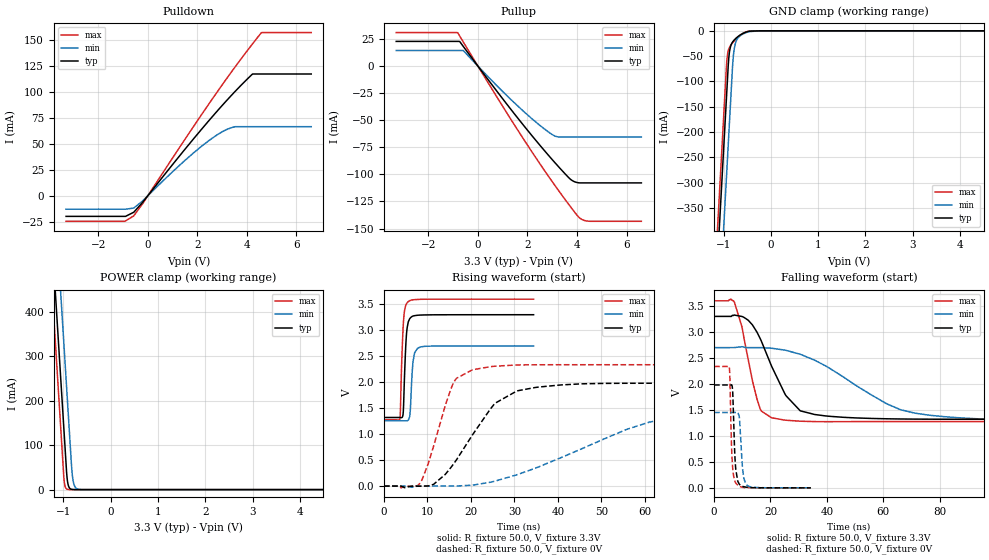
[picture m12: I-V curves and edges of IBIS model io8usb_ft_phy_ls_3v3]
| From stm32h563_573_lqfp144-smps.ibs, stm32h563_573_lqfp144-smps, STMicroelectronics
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[Model]   io8usb_ft_phy_ls_3v3
Model_type I/O
Polarity   Non-Inverting
Enable   Active-Low
| CAP_THRESHOLD on pad DPFT is "UDTCAPC" :
| Rising=20.0% of vddiom   Falling=80.0% of vddiom
| C_comp min and max val. don't necessarily correlate with the min and max pvt
| but are the smallest and greatest pad capacitance found.
| var   typ   min   max
C_comp   8.88570pF  8.80266pF  8.92058pF
|C_comp_pullup   6.10735pF  5.78805pF  5.62765pF
|C_comp_pulldown   2.77835pF  3.01461pF  3.29293pF
Vinl = 1.35V
Vinh = 1.8V
Vmeas = 1.65V   | Reference voltage for timing measurements
Cref  = 50.0pF   | Timing specification test load capacitance value
Rref  = 1.0MOhm   | Timing specification test load resistance value
Vref  = 1.815V   | Timing specification test load voltage
[Model Spec]
| TIME_THRESHOLD on pin ZIUSBPV11 is "CMOS" :
| Rising=40.0% of vdd   Falling=60.0% of vdd
Vinl 1.31380V 1.08880V 1.42380V
Vinh 1.79320V 1.51020V 1.91620V
| variable   typ   min   max
[Temperature Range] 25.0 125.0 -40.0
| variable   typ   min   max
[Voltage Range] 3.3V 2.7V 3.6V
| variable   typ   min   max
[POWER Clamp Reference] 3.3V 2.7V 3.6V
| variable   typ   min   max
[GND Clamp Reference] 0V 0V 0V
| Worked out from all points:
|   slope of the pulldown table from 0 to 0.495 V, typ, clamps not added: 33.1 ohm
|   slope of the pullup table from 0 to 0.495 V, typ, clamps not added: 32.9 ohm
|   GND clamp passes 1 mA (typ) near -0.46 V on its own axis
|   POWER clamp passes 1 mA (typ) near -0.84 V on its own axis
|   rising waveform, R_fixture 50.0, V_fixture 3.3V: 20-80 % time 589ps typ, 600ps min, 595ps max; typ from 1.32 V to 3.3 V
|   falling waveform, R_fixture 50.0, V_fixture 3.3V: 20-80 % time 10.4ns typ, 27.1ns min, 5.39ns max; typ from 3.3 V to 1.32 V
|   rising waveform, R_fixture 50.0, V_fixture 0V: 20-80 % time 9.68ns typ, 25.4ns min, 5.08ns max; typ from 0 V to 1.98 V
|   falling waveform, R_fixture 50.0, V_fixture 0V: 20-80 % time 860ps typ, 1.08ns min, 778ps max; typ from 1.98 V to 0 V
[POWER Clamp]
-3.3V     4.068A     4.259A     3.957A
-1.25V    582.8mA    774.2mA    471.5mA
-1.16V    429.8mA    621.2mA    318.5mA
-1.05V    242.8mA    434.2mA    131.5mA
-980mV    123.8mA    315.2mA    17.95mA
-960mV    89.81mA    281.2mA    6.634mA
-920mV    26.3mA     213.2mA    906uA
-880mV    5.543mA    145.2mA    123.7uA
-810mV    363.5uA    33.6mA     3.798uA
-770mV    76.63uA    10.47mA    519.9nA
-690mV    3.411uA    1.017mA    10.89nA
6.6V      0A         0A         0A
[GND Clamp]
-3.3V     -4.147A    -4.304A    -4.084A
-1.25V    -662.3mA   -818.9mA   -599mA
-940mV    -135.3mA   -291.9mA   -71.97mA
-910mV    -84.3mA    -240.9mA   -43.19mA
-890mV    -54.53mA   -206.9mA   -36.04mA
-870mV    -38.95mA   -172.9mA   -31.83mA
-810mV    -22.29mA   -70.86mA   -23.78mA
-780mV    -18.66mA   -39.68mA   -20.49mA
-750mV    -15.77mA   -25.18mA   -17.46mA
-710mV    -12.47mA   -16.15mA   -13.75mA
-540mV    -3.025mA   -4.157mA   -2.753mA
6.6V      24.07nA    4.253uA    975.9pA
| variable   typ   min   max
[Pullup Reference] 3.3V 2.7V 3.6V
| variable   typ   min   max
[Pulldown Reference] 0V 0V 0V
[Pullup]
-3.3V     22.83mA    14.39mA    31mA
-820mV    22.83mA    14.39mA    31mA
-740mV    22.83mA    14.39mA    27.95mA
-590mV    18.16mA    14.39mA    22.24mA
1.32V     -39.61mA   -30.57mA   -48.77mA
2.85V     -82.4mA    -60.84mA   -101.8mA
3.19V     -91.23mA   -65.16mA   -112.8mA
3.7V      -103.7mA   -65.39mA   -128.7mA
4.06V     -107.7mA   -65.39mA   -139.2mA
4.22V     -107.9mA   -65.39mA   -141.9mA
4.51V     -107.9mA   -65.39mA   -143.3mA
6.6V      -107.9mA   -65.39mA   -143.3mA
[Pulldown]
-3.3V     -19.88mA   -12.95mA   -24.65mA
-940mV    -19.88mA   -12.95mA   -24.65mA
-570mV    -15.96mA   -11.9mA    -19.44mA
-220mV    -6.69mA    -5.247mA   -8.037mA
1.48V     44.27mA    33.69mA    53.76mA
2.17V     64.17mA    47.77mA    78.28mA
2.8V      81.66mA    58.79mA    100.1mA
3.19V     92.07mA    63.96mA    113.3mA
3.51V     100.3mA    66.56mA    123.9mA
4.23V     117.5mA    66.66mA    146.6mA
4.59V     117.5mA    66.66mA    157.5mA
6.6V      117.5mA    66.66mA    157.5mA
[Ramp]
dV/dt_r 1.18821V/9.67363ns 870.42399mV/24.97673ns 1.40193V/5.07203ns
dV/dt_f 1.18779V/10.0041ns 865.87422mV/26.69286ns 1.3938V/5.29566ns
R_load = 50.0
| Removed startup time: 0s 0s 0s  .
| Removed end time: 34.4ns.
[Rising Waveform]
R_fixture   = 50.0
V_fixture   = 3.3V
V_fixture_min = 2.7V
V_fixture_max = 3.6V
0s        1.32V      1.257V     1.277V
3.65ns    1.32V      1.257V     1.288V
3.75ns    1.32V      1.257V     1.376V
4.5ns     1.521V     1.257V     3.181V
5.05ns    2.754V     1.257V     3.486V
5.6ns     3.163V     1.268V     3.553V
6ns       3.232V     1.396V     3.573V
6.7ns     3.275V     2.404V     3.587V
7.75ns    3.29V      2.656V     3.594V
34.4ns    3.3V       2.7V       3.6V
| Removed startup time: 0s 0s 0s  .
| Removed end time: 249.35ns.
[Falling Waveform]
R_fixture   = 50.0
V_fixture   = 3.3V
V_fixture_min = 2.7V
V_fixture_max = 3.6V
0s        3.3V       2.7V       3.6V
7.2ns     3.326V     2.7V       3.575V
9.9ns     3.298V     2.717V     3.096V
12.2ns    3.221V     2.699V     2.444V
16.75ns   2.826V     2.699V     1.478V
25ns      1.821V     2.652V     1.304V
35.65ns   1.412V     2.458V     1.276V
61.1ns    1.33V      1.621V     1.277V
76.35ns   1.322V     1.398V     1.277V
249.3ns   1.32V      1.257V     1.277V
| Removed startup time: 0s 0s 0s  .
| Removed end time: 249.4ns.
[Rising Waveform]
R_fixture   = 50.0
V_fixture   = 0V
V_fixture_min = 0V
V_fixture_max = 0V
0s        24.82nV    1.065uV    39.76nV
8.1ns     -1.878mV   -1.788mV   37.66mV
11.4ns    31.98mV    -774.9uV   764.2mV
16.2ns    449.3mV    472.3uV    2.017V
24.4ns    1.476V     72.49mV    2.298V
30.6ns    1.833V     218.2mV    2.332V
35.6ns    1.907V     370.6mV    2.336V
61.1ns    1.98V      1.233V     2.337V
75.3ns    1.98V      1.376V     2.337V
249.4ns   1.98V      1.451V     2.337V
| Removed startup time: 0s 0s 0s  .
| Removed end time: 34.35ns.
[Falling Waveform]
R_fixture   = 50.0
V_fixture   = 0V
V_fixture_min = 0V
V_fixture_max = 0V
0s        1.98V      1.451V     2.337V
5.35ns    1.98V      1.451V     2.329V
5.6ns     1.98V      1.451V     2.125V
6.05ns    1.981V     1.451V     1.052V
6.4ns     1.958V     1.451V     546.4mV
7.7ns     352.2mV    1.451V     91.95mV
8.9ns     74.21mV    1.381V     33.24mV
10.1ns    29.35mV    365.7mV    10.98mV
11.25ns   14.26mV    73.13mV    3.146mV
34.35ns   162.6uV    421.2uV    147.6uV
